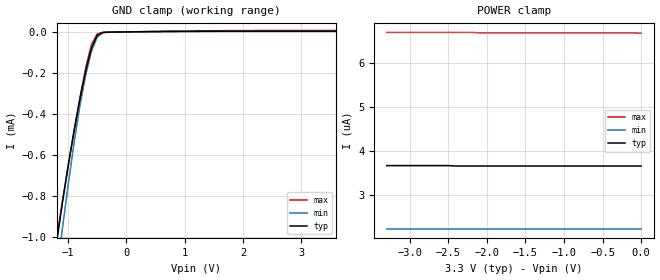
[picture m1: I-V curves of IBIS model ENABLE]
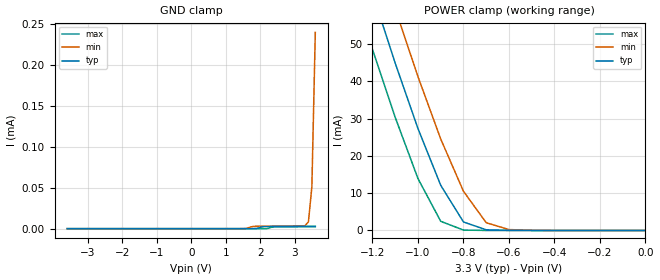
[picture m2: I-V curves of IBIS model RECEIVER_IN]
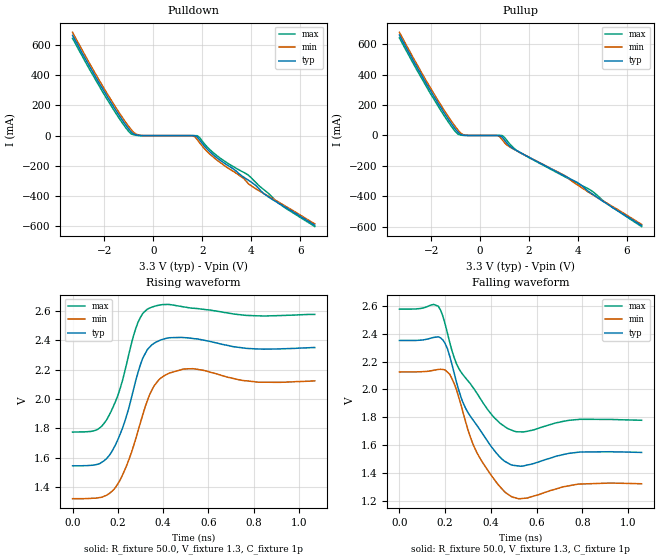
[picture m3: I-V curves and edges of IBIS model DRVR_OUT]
|   Texas Instruments Incorporated
|   Data Transmissions Products
|   IBIS Model for SN65LVP20
|   8DRF  Small-Outline No-Lead Package
[IBIS Ver]   3.2
[Comment char]   |_char
[File name]   lvp20.ibs
[File Rev]   1.1
[Date]   24May04
[Source]   File originated at Texas Instruments Incorporated.
   Data Transmission Products Group.
[Notes]
[Disclaimer]
(C) Copyright Texas Instruments Incorporated 2004
   All rights reserved
  Texas Instruments Incorporated hereby grants the user of this IBIS
model a non-exclusive, nontransferable license to use this IBIS model
under the following terms.  Before using this IBIS model, the user
should read this license.  If the user does not accept these terms,
the IBIS model should be returned to Texas Instruments within 30 days.
  The user is granted this license only to use the IBIS model and
is not granted rights to sell, load, rent, lease or license the IBIS
model in whole or in part, or in modified form to anyone other than
user.  User may modify the IBIS model to suit its specific applications
but rights to derivative works and such modifications shall belong to
Texas Instruments.
  This IBIS model is provided on an "AS IS" basis and Texas Instruments
makes absolutely no warranty with respect to the information contained
herein.  TEXAS INSTRUMENTS DISCLAIMS AND CUSTOMER WAIVES ALL WARRANTIES,
EXPRESS OR IMPLIED, INCLUDING WARRANTIES OF MERCHANTABILITY OR FITNESS
FOR A PARTICULAR PURPOSE. The entire risk as to quality and performance
is with the Customer. ACCORDINGLY, IN NO EVENT SHALL THE COMPANY BE LIABLE
FOR ANY DAMAGES, WHETHER IN CONTRACT OR TORT,INCLUDING ANY LOST PROFITS
OR OTHER INCIDENTAL, CONSEQUENTIAL, EXEMPLARY, OR PUNITIVE DAMAGES ARISING
OUT OF THE USE OR APPLICATION OF THE IBIS model provided in this package.
Further, Texas Instruments reserves the right to discontinue or make changes
without notice to any product herein to improve reliability, function, or
design. Texas Instruments does not convey any license under patent rights
or any other intellectual property rights, including those of third parties.
Contact Texas Instruments at ATTN:DATA TRANSMISSIONS
[Copyright]   Copyright 2004, Texas Instruments, All Rights Reserved
[Component]   LVP20DRF
[Manufacturer]  Texas Instruments Incorporated
[Package]
|   typ   min   max
R_pkg   0.189   0.176   0.203
L_pkg   0.802nH   0.759nH   0.850nH
C_pkg   0.053pF   0.046pF   0.067pF
[Pin]   signal_name   model_name   R_pin   L_pin   C_pin
1   NC   NC   0.194   0.817n   0.054p
2   A   RECEIVER_IN   0.193   0.814n   0.054p
3   B   RECEIVER_IN   0.187   0.793n   0.052p
4   VBB   POWER   0.194   0.821n   0.054p
5   EN/   ENABLE   0.176   0.759n   0.046p
6   Z   DRVR_OUT   0.188   0.799n   0.051p
7   Y   DRVR_OUT   0.181   0.772n   0.050p
8   VCC   POWER   0.187   0.791n   0.052p
9   GND   GND   0.203   0.850n   0.067p
[Diff_pin]   inv_pin   vdiff   tdelay_typ   tdelay_min   tdelay_max
| The 'A/Y' pin is Diff_pin and the 'B/Z' pin is the inv_pin
2   3   0.100   0 0 0
7   6   0.000   0 0 0
| Models and submodels in the file (3): ENABLE (Input), RECEIVER_IN (Input), DRVR_OUT (Output_ECL)
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|   Enable Input Model
[Model]   ENABLE
Model_type   Input
|Signals   /E
Vinh = 2.0
Vinl = 0.8
C_comp   3.3pF   3.28pF   3.38pF
|   typ   min   max
[Temperature Range]   25   -40   85
[Voltage range]   3.3V   3.0V   3.6V
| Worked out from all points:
|   GND clamp passes 1 mA (typ) near -1.18 V on its own axis
[GND_clamp]
|Voltage I(typ)   I(min)   I(max)
-3.6V     -6.81mA    -7.03mA    -6.59mA
-1.2V     -1.03mA    -1.18mA    -1.01mA
-1.1V     -834uA     -961uA     -829uA
-1V       -652uA     -745uA     -654uA
-900mV    -485uA     -543uA     -484uA
-800mV    -330uA     -362uA     -323uA
-700mV    -191uA     -211uA     -176uA
-600mV    -78.2uA    -93.9uA    -60.7uA
-500mV    -15.7uA    -24.3uA    -8.94uA
-400mV    -2.37uA    -3.64uA    -2.58uA
-300mV    -1.1uA     -901nA     -1.79uA
3.6V      3.66uA     2.24uA     6.67uA
[Power_clamp]
| Note that the[POWER_clamp]voltage table is referenced to Vcc
| and is calculated using Vtable=Vcc - Vmeasured.
|Voltage I(typ)   I(min)   I(max)
-3.3V     3.67uA     2.24uA     6.69uA
-2.5V     3.67uA     2.24uA     6.69uA
-2.4V     3.66uA     2.24uA     6.69uA
-2.2V     3.66uA     2.24uA     6.69uA
-2.1V     3.66uA     2.24uA     6.68uA
-100mV    3.66uA     2.24uA     6.68uA
0V        3.66uA     2.24uA     6.67uA
|   Receiver Input Model
[Model]   RECEIVER_IN
Model_type   Input
|Signals   A, B
Vinh = 2.2
Vinl = 1.8
|   typ   min   max
C_comp   1.0pF   0.98pF   1.10pF
|   typ   min   max
[Temperature Range]   25   -40   85
[Voltage range]   3.3V   3.0V   3.6V
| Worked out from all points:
|   POWER clamp passes 1 mA (typ) near -0.74 V on its own axis
[GND_clamp]
|Voltage I(typ)   I(min)   I(max)
-3.6V     -93.5pA    -92.3pA    -96.3pA
1.5V      -4.04pA    13.2nA     -8.24pA
1.8V      4.55nA     2.8uA      -3.22pA
2.1V      2.52uA     3.01uA     483pA
2.4V      2.64uA     3.1uA      2.1uA
3.3V      2.9uA      3.61uA     2.32uA
3.4V      2.93uA     8.35uA     2.35uA
3.5V      2.96uA     51uA       2.37uA
3.6V      2.99uA     240uA      2.4uA
[Power_clamp]
| Note that the[POWER_clamp]voltage table is referenced to Vcc
| and is calculated using Vtable=Vcc - Vmeasured.
|Voltage   I(typ)   I(min)   I(max)
-3.3V     557mA      575mA      539mA
-1.3V     83.2mA     98.5mA     67.8mA
-1.2V     63.6mA     78.6mA     48.5mA
-1.1V     44.8mA     59.4mA     30.3mA
-1V       27.3mA     41.2mA     13.9mA
-900mV    12.1mA     24.5mA     2.46mA
-800mV    2.28mA     10.5mA     111uA
-700mV    181uA      2.08mA     10.4uA
-600mV    29.5uA     240uA      2.64uA
0V        2.9uA      3.29uA     2.4uA
|   Driver Output Model
[Model]   DRVR_OUT
Model_type   Output_ECL
| Signals   Y,Z
Vmeas = 2.0V   |Reference voltage for timing measurements
Cref = 0pF   |Timing specification test load capacitance value
Rref = 50
|Note: 50 Ohm load; single ended configuration
| variable   typ   min   max
C_comp   0.8pF   0.6pF   0.9pF
|   typ   min   max
[Temperature Range]   25   -40   85
[Voltage range]   3.3V   3.0V   3.6V
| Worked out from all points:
|   rising waveform, R_fixture 50.0, V_fixture 1.3, C_fixture 1p: 20-80 % time 95.7ps typ, 104ps min, 90.8ps max; typ from 1.54 V to 2.35 V
|   falling waveform, R_fixture 50.0, V_fixture 1.3, C_fixture 1p: 20-80 % time 125ps typ, 105ps min, 144ps max; typ from 2.35 V to 1.55 V
[Pulldown]
|Voltage I(typ)   I(min)   I(max)
| Note that the[Pulldown]voltage table for (P)ECL is referenced
| to Vcc and is calculated using Vtable=Vcc - Vmeasured.
-3.3V     665mA      685mA      645mA
-1.6V     185mA      204mA      166mA
-1V       43mA       59.7mA     26.4mA
-800mV    10.5mA     21.4mA     5.1mA
-400mV    4.63uA     184uA      6.49nA
1.6V      -13.8uA    -610uA     -49.5nA
1.8V      -9.83mA    -27mA      -827uA
2.6V      -147mA     -162mA     -133mA
3.7V      -276mA     -285mA     -244mA
3.9V      -297mA     -321mA     -264mA
5.1V      -446mA     -439mA     -446mA
6.6V      -594mA     -585mA     -603mA
[Pullup]
|Voltage   I(typ)   I(min)   I(max)
| Note that the[Pullup]voltage table is referenced to Vcc
| and is calculated using Vtable=Vcc - Vmeasured.
-3.3V     660mA      678mA      641mA
-1.6V     181mA      198mA      162mA
-1V       38.9mA     54.4mA     22.9mA
-800mV    6.8mA      16.6mA     2.2mA
-600mV    174uA      993uA      1.73uA
700mV     -17.7uA    -731uA     -46.4nA
900mV     -10.8mA    -27.6mA    -775uA
1.2V      -69.4mA    -74.7mA    -54.2mA
1.5V      -100mA     -101mA     -99.8mA
3.5V      -270mA     -268mA     -275mA
4.5V      -376mA     -380mA     -358mA
6.6V      -593mA     -585mA     -599mA
[Ramp]
|   typ   min   max
dV/dt_r   0.484/92ps   0.482/105ps   0.481/90ps
dV/dt_f   0.482/90ps   0.482/105ps   0.479/145ps
R_load = 50ohm  |Note: The measurement is with 50ohm to Vtt.
[Rising Waveform]
R_fixture = 50.0
V_fixture = 1.3
V_fixture_min = 1.0
V_fixture_max = 1.6
C_fixture = 1p
L_fixture = 0n
|   V(typ)  V(min)  V(max)
0s        1.545V     1.321V     1.775V
120ps     1.56V      1.329V     1.803V
190ps     1.689V     1.398V     1.985V
240ps     1.893V     1.551V     2.248V
280ps     2.131V     1.733V     2.485V
340ps     2.353V     2.028V     2.62V
390ps     2.403V     2.143V     2.642V
490ps     2.419V     2.204V     2.628V
820ps     2.341V     2.115V     2.567V
1.07ns    2.351V     2.124V     2.577V
[Falling Waveform]
R_fixture = 50.0
V_fixture = 1.3
V_fixture_min = 1.0
V_fixture_max = 1.6
C_fixture = 1p
L_fixture = 0n
|   V(typ)  V(min)  V(max)
0s        2.352V     2.126V     2.577V
170ps     2.378V     2.144V     2.598V
220ps     2.24V      2.11V      2.339V
250ps     2.05V      1.996V     2.183V
280ps     1.899V     1.825V     2.102V
340ps     1.74V      1.543V     1.971V
410ps     1.573V     1.365V     1.807V
490ps     1.458V     1.231V     1.709V
790ps     1.551V     1.321V     1.786V
1.06ns    1.548V     1.323V     1.779V
